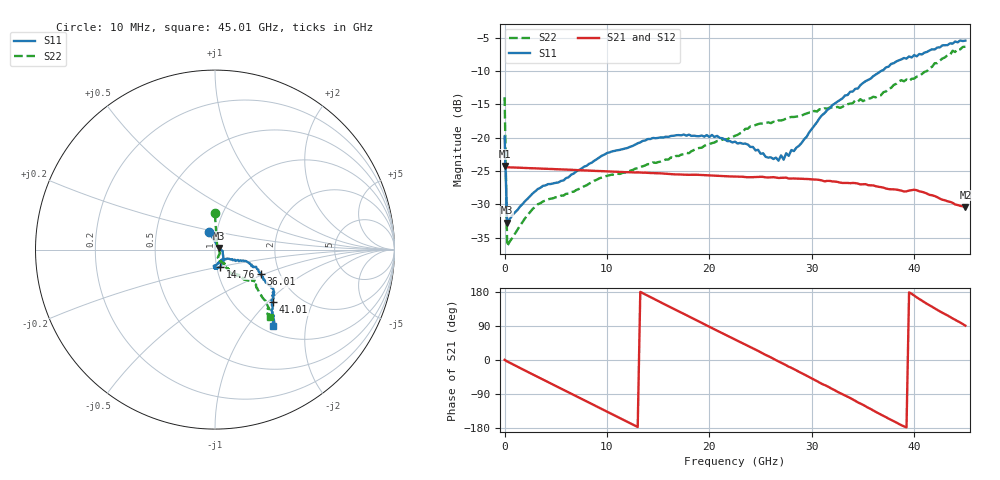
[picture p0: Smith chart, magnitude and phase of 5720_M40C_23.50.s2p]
! Device:  ADRF5720
! Description: 0.5dB LSB GaAs MMIC 6-bit Digital Attenuator
! Frequency:  0.000009 -  40 GHz
! Ports:
!	RF1	= Port 1
!	RF2	= Port 2
! Vdd:  3.3 Volt
! Vss:  -3.3 Volt
! Control:  0/3.3 Volt
! State:  23.50 dB attenuation
! Data:  The device was measured using G-S-G Probes on a matrix board.
!  Data was collected using an calibrated 4 port network analyzer.
!  The reference plane for this measurement is at the launchers.
! Note:  Analog Devices supplies this data as a sample of measured data
!  for this product.  Your particular data for this product may vary.
!  Data was taken at -40 degrees C.
!  Analog Devices reserves the right to change this data at anytime.
# GHZ S DB R 45.0
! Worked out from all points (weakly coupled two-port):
!   181 points, 10 MHz to 45.01 GHz, reference 45 ohm
!   highest |S21| = -24.24 dB at 10 MHz (marker M1); lowest = -30.4 dB at 45.01 GHz (marker M2)
!   lowest |S11| = -32.7 dB at 260 MHz (marker M3), VSWR 1.05, Z = 46.9 + j0.881 ohm
!   |S11| at or under -10 dB: start of sweep to 36.75 GHz
!   |S22| runs from -36.2 to -6.3 dB; largest |S21 - S12| = 0.0003
!   S11 on the Smith chart (normalised r, x): 10 MHz: 0.92, +0.18; 14.76 GHz: 1.04, -0.20; 36.01 GHz: 1.61, -0.47; 41.01 GHz: 1.49, -1.07; 45.01 GHz: 1.12, -1.34
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0.01  -19.81 108.7  -24.24 0.4  -24.27 0.4  -13.92 90.3
0.26  -32.73 24.0  -24.42 -3.8  -24.44 -3.8  -36.25 32.4
3.26  -27.67 -9.9  -24.60 -44.9  -24.62 -44.9  -29.96 -32.0
5.76  -26.40 -26.1  -24.75 -78.7  -24.77 -78.7  -28.66 -51.8
7.76  -24.34 -40.6  -24.88 -105.8  -24.90 -105.8  -27.28 -65.7
10.01  -22.28 -51.5  -25.03 -136.2  -25.05 -136.2  -25.70 -70.2
14.76  -20.06 -73.4  -25.31 159.1  -25.33 159.0  -23.76 -68.2
15.26  -19.93 -75.5  -25.33 152.1  -25.35 152.1  -23.56 -67.9
20.26  -19.57 -91.2  -25.66 84.2  -25.68 84.2  -20.81 -58.5
22.76  -20.86 -94.0  -25.83 50.7  -25.85 50.6  -19.56 -58.6
24.01  -21.37 -85.0  -25.91 34.2  -25.93 34.1  -18.29 -57.6
25.51  -22.86 -71.3  -25.93 13.3  -25.95 13.2  -17.79 -55.9
26.76  -23.42 -57.7  -26.02 -3.6  -26.03 -3.8  -17.38 -55.6
27.01  -22.63 -54.4  -26.00 -6.8  -26.02 -7.0  -17.39 -57.1
27.26  -23.28 -53.4  -25.99 -10.4  -26.01 -10.5  -17.30 -55.5
30.26  -18.17 -27.0  -26.25 -52.1  -26.27 -52.2  -15.96 -56.8
32.01  -15.10 -21.4  -26.54 -76.5  -26.57 -76.6  -15.49 -53.4
36.01  -10.76 -27.6  -27.14 -133.2  -27.16 -133.4  -13.84 -47.0
37.76  -8.91 -33.5  -27.72 -157.8  -27.75 -158.0  -12.51 -45.1
41.01  -7.22 -42.0  -28.21 152.2  -28.25 152.1  -10.12 -42.6
43.76  -5.88 -49.9  -29.75 109.6  -29.78 109.4  -6.94 -47.6
45.01  -5.42 -52.8  -30.39 90.7  -30.42 90.5  -6.34 -50.9
